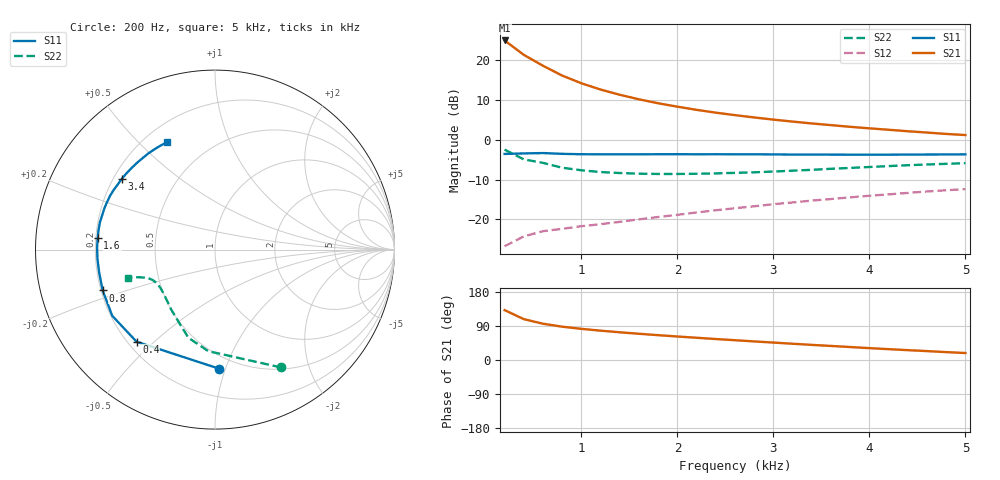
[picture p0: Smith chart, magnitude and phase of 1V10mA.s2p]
#  HZ  S  MA  R  50.0000
! Device:MCH4020
! Bias:VCE=1V, IC=10mA
!MHZ	S11(MAG/ANG)		S21(MAG/ANG)		S12(MAG/ANG)		S22(MAG/ANG)
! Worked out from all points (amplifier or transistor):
!   25 points, 200 Hz to 5 kHz, reference 50 ohm
!   highest |S21| = 25.0 dB at 200 Hz (marker M1)
!   |S21| within 3 dB of that: start of sweep to 365.6 Hz
!   unconditionally stable (mu >= 1): 2.239 kHz to end of sweep
!   at 1 kHz: K = 0.62, MSG = 18.0 dB, |S12| = -21.7 dB
!   at 2.6 kHz: K = 1.03, MAG = 10.6 dB, |S12| = -17.2 dB
!   at 5 kHz: K = 1.00, MAG = 6.6 dB, |S12| = -12.4 dB
!   S11 on the Smith chart (normalised r, x): 200 Hz: 0.40, -0.95; 400 Hz: 0.23, -0.44; 800 Hz: 0.21, -0.17; 1.6 kHz: 0.21, +0.05; 3.4 kHz: 0.23, +0.32; 5 kHz: 0.29, +0.61
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200  0.664 -88.0  17.73 131.6  0.046 52.6  0.753 -60.7
400  0.674 -130.4  11.68 107.8  0.061 40.5  0.567 -93.8
600  0.681 -147.2  8.523 95.7  0.071 38.0  0.513 -106.8
800  0.666 -160.0  6.411 87.9  0.076 38.4  0.445 -118.0
1000  0.658 -168.7  5.131 82.2  0.082 39.7  0.414 -126.1
1200  0.657 -175.3  4.28 77.4  0.087 41.3  0.393 -132.2
1400  0.657 179.2  3.679 73.1  0.093 42.8  0.382 -136.8
1600  0.657 174.3  3.228 69.2  0.1 44.4  0.375 -141.0
1800  0.658 170.2  2.878 65.5  0.107 45.5  0.372 -143.9
2000  0.659 166.6  2.608 62.0  0.114 46.5  0.372 -146.8
2200  0.657 162.8  2.379 58.7  0.122 47.2  0.374 -149.0
2400  0.658 159.4  2.193 55.3  0.13 47.6  0.378 -151.2
2600  0.657 156.0  2.041 52.2  0.138 47.8  0.384 -153.4
2800  0.657 152.7  1.909 49.0  0.146 47.9  0.39 -154.6
3000  0.655 149.4  1.793 46.0  0.155 47.8  0.399 -156.0
3200  0.652 146.0  1.693 42.9  0.163 47.5  0.409 -157.2
3400  0.652 142.6  1.605 39.9  0.172 47.1  0.419 -158.1
3800  0.65 135.6  1.456 34.2  0.189 45.8  0.443 -159.6
4000  0.65 131.8  1.393 31.3  0.198 45.0  0.455 -160.2
4200  0.65 128.2  1.337 28.6  0.206 44.2  0.467 -160.8
4800  0.654 117.3  1.185 20.8  0.232 41.1  0.499 -161.7
5000  0.656 113.8  1.147 18.4  0.24 40.0  0.508 -162.1
